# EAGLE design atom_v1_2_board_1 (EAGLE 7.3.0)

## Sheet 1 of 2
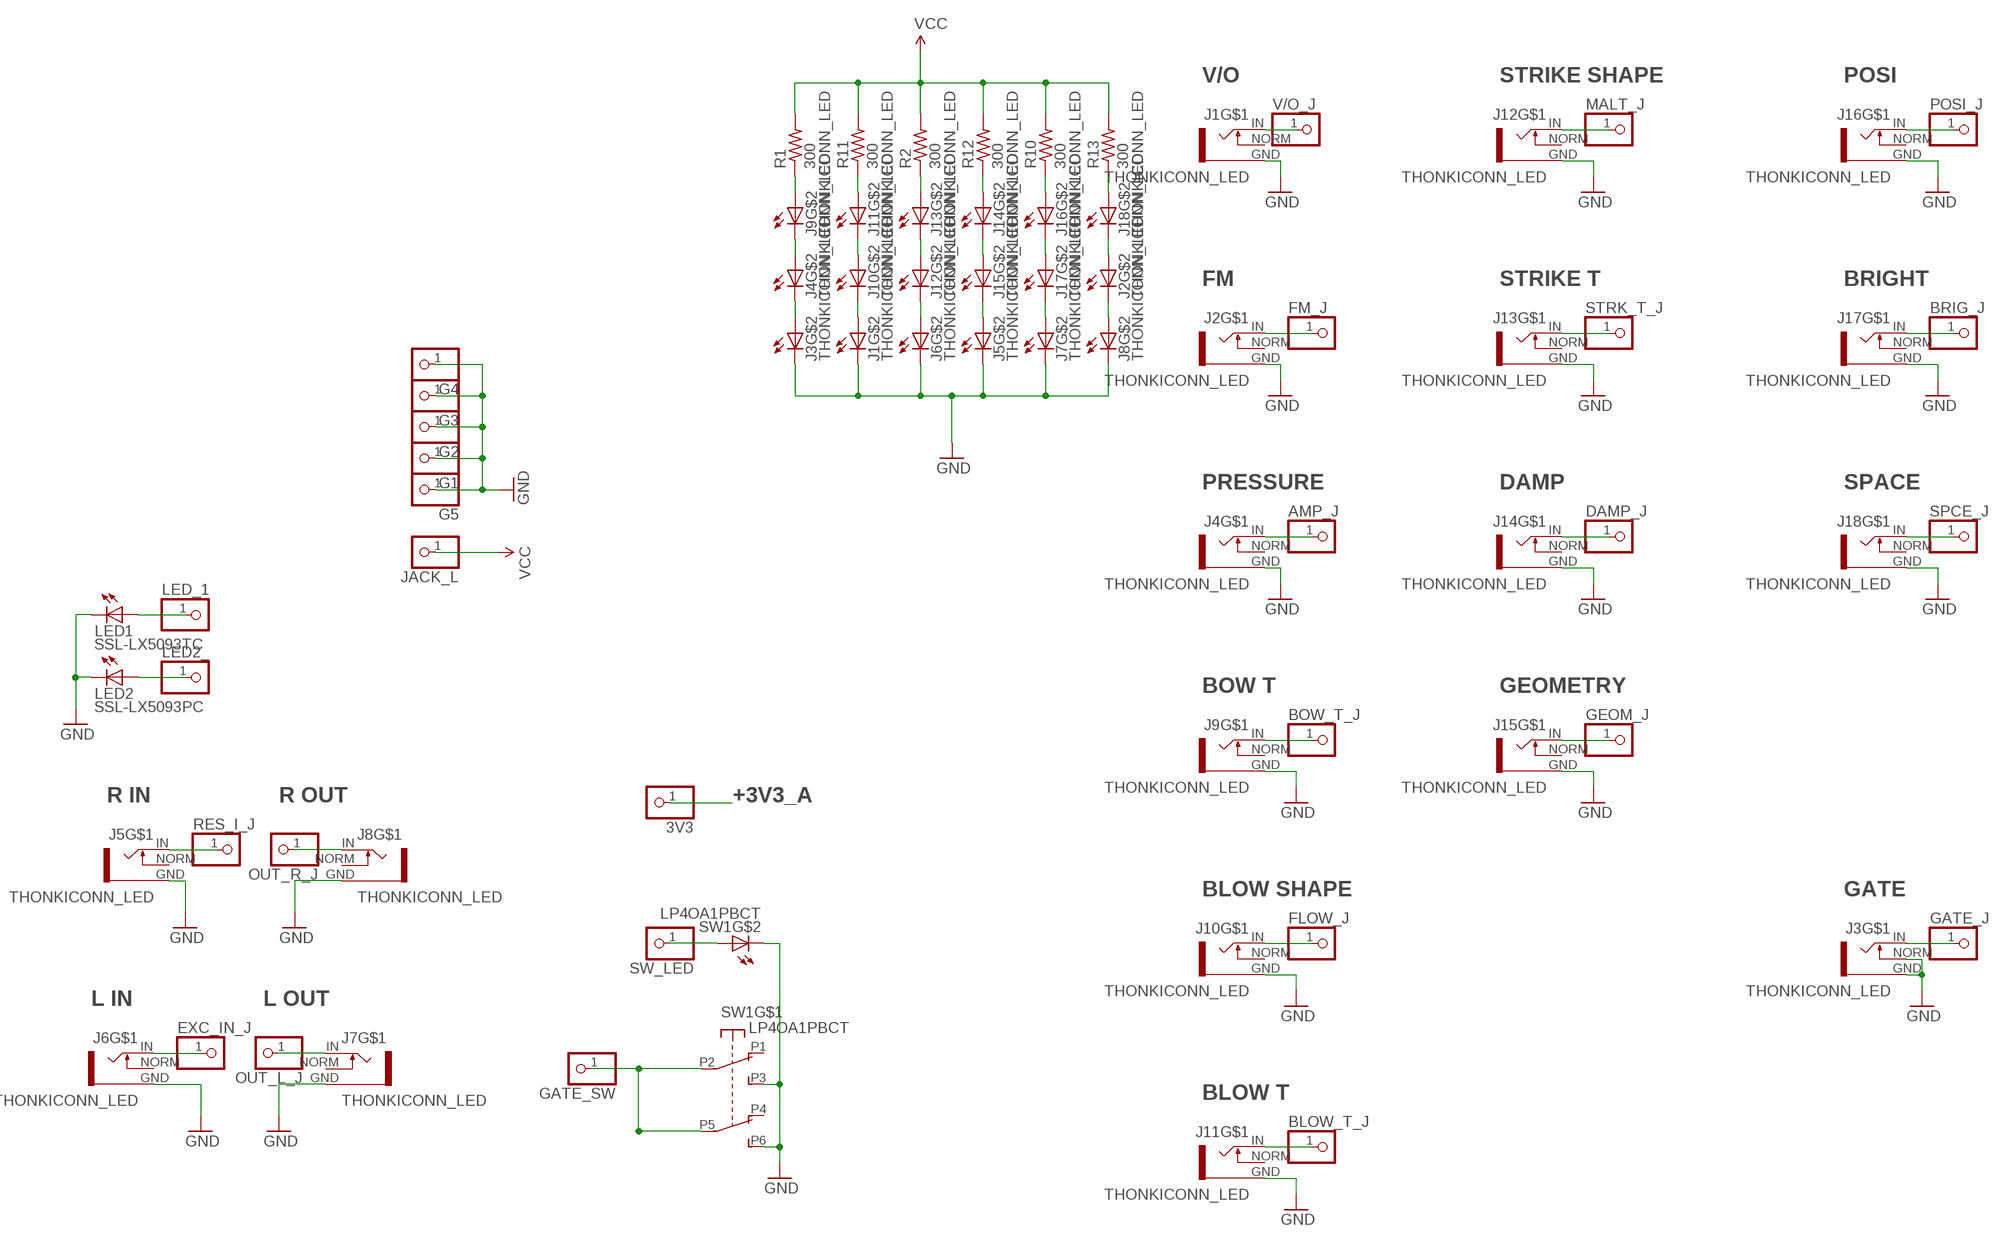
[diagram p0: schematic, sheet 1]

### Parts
3V3  PINHD-1X1  [1X01]
AMP_J  PINHD-1X1  [1X01]
BLOW_T_J  PINHD-1X1  [1X01]
BOW_T_J  PINHD-1X1  [1X01]
BRIG_J  PINHD-1X1  [1X01]
DAMP_J  PINHD-1X1  [1X01]
EXC_IN_J  PINHD-1X1  [1X01]
FLOW_J  PINHD-1X1  [1X01]
FM_J  PINHD-1X1  [1X01]
G1  PINHD-1X1  [1X01]
G2  PINHD-1X1  [1X01]
G3  PINHD-1X1  [1X01]
G4  PINHD-1X1  [1X01]
G5  PINHD-1X1  [1X01]
GATE_J  PINHD-1X1  [1X01]
GATE_SW  PINHD-1X1  [1X01]
GEOM_J  PINHD-1X1  [1X01]
J1  THONKICONN_LED  [LED_JACK]
J2  THONKICONN_LED  [LED_JACK]
J3  THONKICONN_LED  [LED_JACK]
J4  THONKICONN_LED  [LED_JACK]
J5  THONKICONN_LED  [LED_JACK]
J6  THONKICONN_LED  [LED_JACK]
J7  THONKICONN_LED  [LED_JACK]
J8  THONKICONN_LED  [LED_JACK]
J9  THONKICONN_LED  [LED_JACK]
J10  THONKICONN_LED  [LED_JACK]
J11  THONKICONN_LED  [LED_JACK]
J12  THONKICONN_LED  [LED_JACK]
J13  THONKICONN_LED  [LED_JACK]
J14  THONKICONN_LED  [LED_JACK]
J15  THONKICONN_LED  [LED_JACK]
J16  THONKICONN_LED  [LED_JACK]
J17  THONKICONN_LED  [LED_JACK]
J18  THONKICONN_LED  [LED_JACK]
JACK_L  PINHD-1X1  [1X01]
LED1  SSL-LX5093TC  LED5MM  [LED_5MM]
LED2  SSL-LX5093PC  LED5MM  [LED_5MM]
LED2_  PINHD-1X1  [1X01]
LED_1  PINHD-1X1  [1X01]
MALT_J  PINHD-1X1  [1X01]
OUT_L_J  PINHD-1X1  [1X01]
OUT_R_J  PINHD-1X1  [1X01]
POSI_J  PINHD-1X1  [1X01]
R1  300  RESISTOR  [RESISTOR_0603]
R2  300  RESISTOR  [RESISTOR_0603]
R10  300  RESISTOR  [RESISTOR_0603]
R11  300  RESISTOR  [RESISTOR_0603]
R12  300  RESISTOR  [RESISTOR_0603]
R13  300  RESISTOR  [RESISTOR_0603]
RES_I_J  PINHD-1X1  [1X01]
SPCE_J  PINHD-1X1  [1X01]
STRK_T_J  PINHD-1X1  [1X01]
SW1  LP4OA1PBCT  [LP4OA1PBCT]
SW_LED  PINHD-1X1  [1X01]
V/O_J  PINHD-1X1  [1X01]

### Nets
+3V3_A: 3V3.1 ; also sheet 2
GND: G1.1 G2.1 G3.1 G4.1 G5.1 J1.C J1.GND J2.GND J3.C J3.GND J3.NORM J4.GND J5.C J5.GND J6.C J6.GND J7.C J7.GND J8.C J8.GND J9.GND J10.GND J11.GND J12.GND J13.GND J14.GND J15.GND J16.GND J17.GND J18.GND LED1.K(C) LED2.K(C) SW1.L2 SW1.P3(A3) SW1.P6(B3) ; also sheet 2
N$1: J1.IN V/O_J.1
N$2: J11.A R11.1
N$3: J12.IN MALT_J.1
N$4 [wide]: J9.A R1.1
N$5 [wide]: J4.A J9.C
N$6: FM_J.1 J2.IN
N$7 [wide]: J3.A J4.C
N$8: J10.A J11.C
N$9: J1.A J10.C
N$10: J14.A R12.1
N$11: J14.C J15.A
N$12: J13.IN STRK_T_J.1
N$13: J5.A J15.C
N$14: J18.A R13.1
N$15: J2.A J18.C
N$16: DAMP_J.1 J14.IN
N$17 [wide]: J7.A J17.C
N$18 [wide]: J16.C J17.A
N$19 [wide]: J16.A R10.1
N$20: J5.IN RES_I_J.1
N$21: EXC_IN_J.1 J6.IN
N$22 [wide]: J13.A R2.1
N$23 [wide]: J12.A J13.C
N$24 [wide]: J6.A J12.C
N$25: J2.C J8.A
N$26: AMP_J.1 J4.IN
N$29: J16.IN POSI_J.1
N$34: BRIG_J.1 J17.IN
N$36: GEOM_J.1 J15.IN
N$39: J18.IN SPCE_J.1
N$43: GATE_J.1 J3.IN
N$59: LED1.A LED_1.1
N$60: LED2.A LED2_.1
N$83: J8.IN OUT_R_J.1
N$85: J7.IN OUT_L_J.1
N$90: BOW_T_J.1 J9.IN
N$91: FLOW_J.1 J10.IN
N$92: BLOW_T_J.1 J11.IN
N$128: SW1.L1 SW_LED.1
SW_GATE: GATE_SW.1 SW1.P2(A2) SW1.P5(B2)
VCC [wide]: JACK_L.1 R1.2 R2.2 R10.2 R11.2 R12.2 R13.2
Unconnected: J1.NORM J2.NORM J4.NORM J5.NORM J6.NORM J7.NORM J8.NORM J9.NORM J10.NORM J11.NORM J12.NORM J13.NORM J14.NORM J15.NORM J16.NORM J17.NORM J18.NORM SW1.P1(A1) SW1.P4(B1)

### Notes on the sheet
- V/O | STRIKE SHAPE | POSI
- FM | STRIKE T | BRIGHT
- PRESSURE | DAMP | SPACE
- BOW T | GEOMETRY
- R IN | R OUT
- BLOW SHAPE | GATE
- L IN | L OUT
- BLOW T

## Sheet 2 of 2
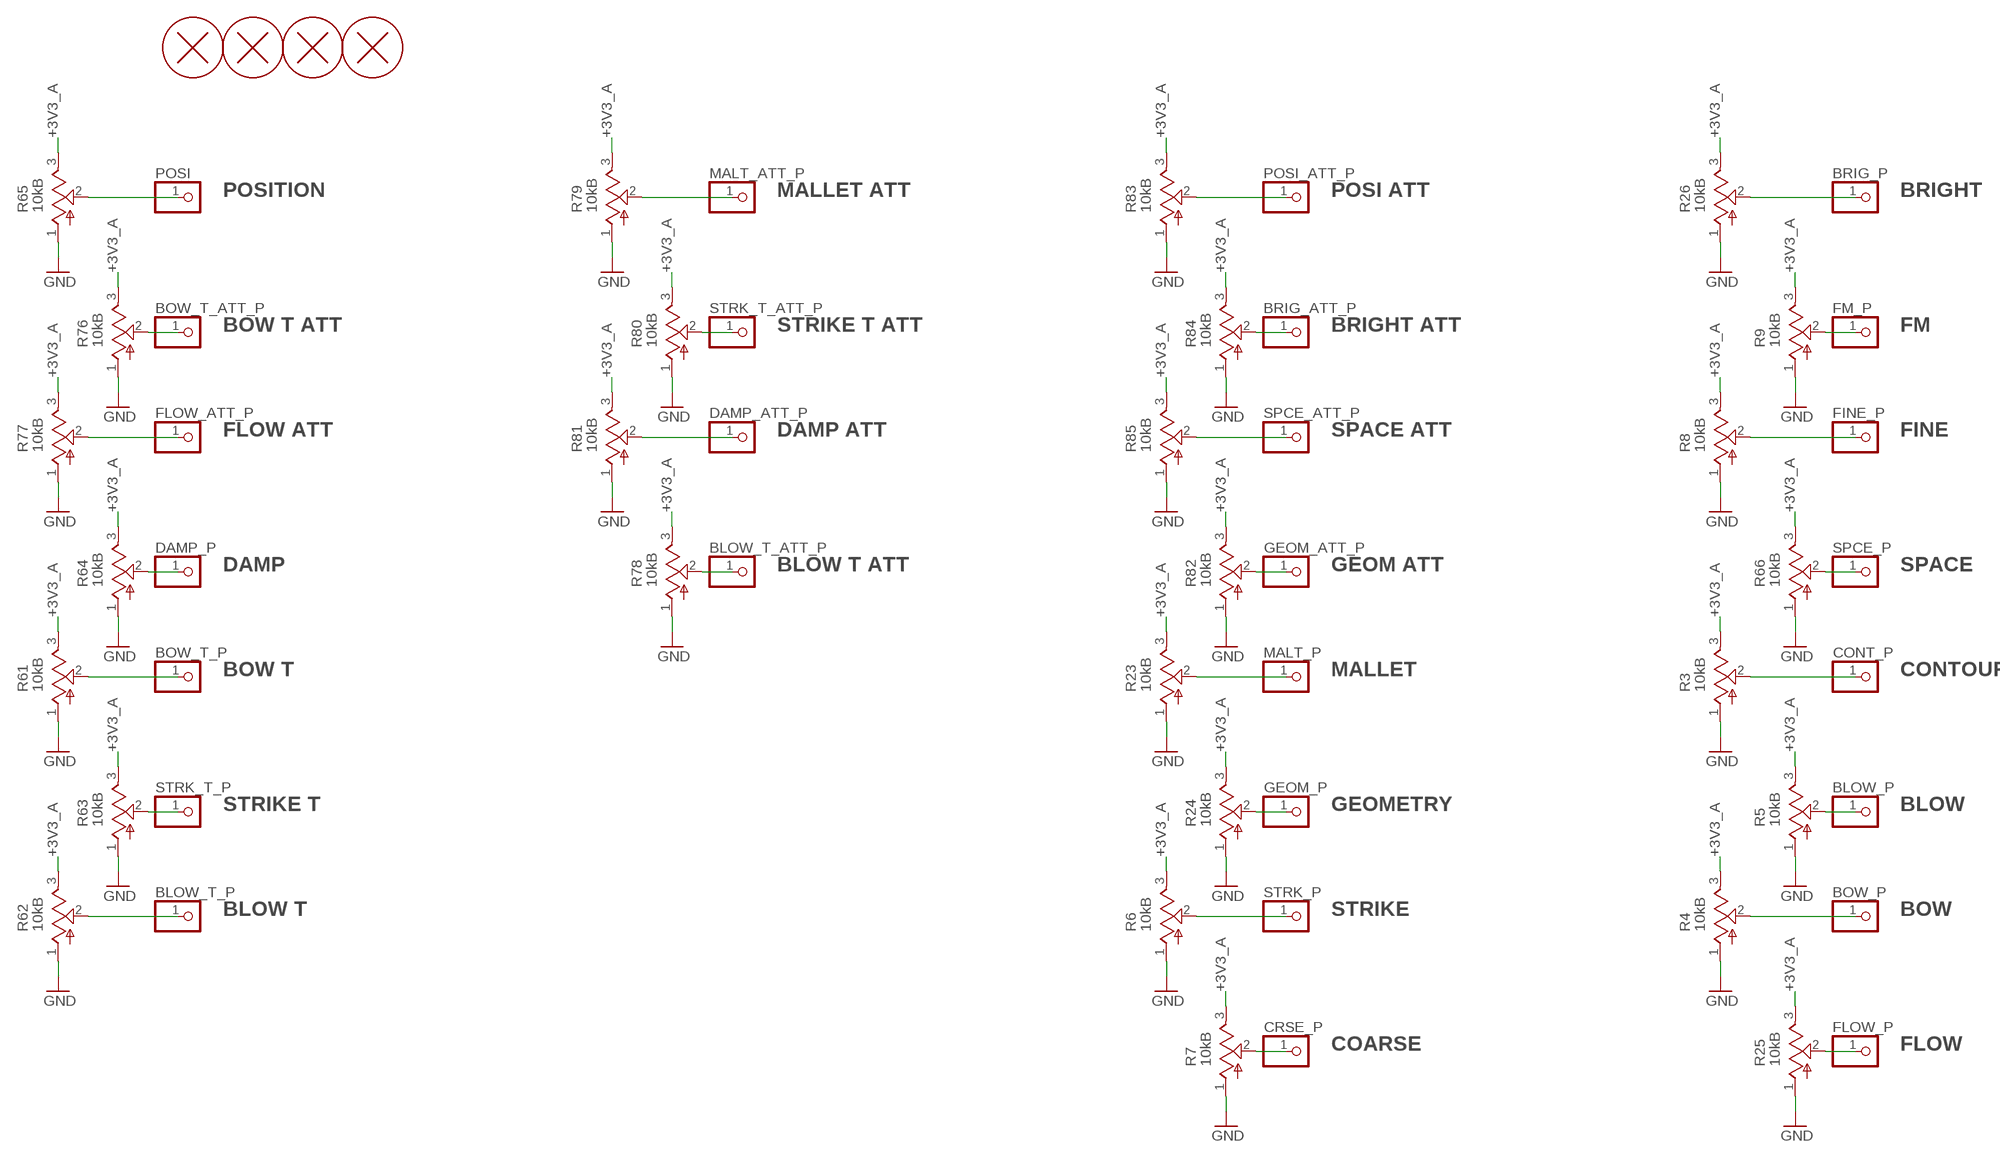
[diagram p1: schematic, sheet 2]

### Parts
BLOW_P  PINHD-1X1  [1X01]
BLOW_T_ATT_P  PINHD-1X1  [1X01]
BLOW_T_P  PINHD-1X1  [1X01]
BOW_P  PINHD-1X1  [1X01]
BOW_T_ATT_P  PINHD-1X1  [1X01]
BOW_T_P  PINHD-1X1  [1X01]
BRIG_ATT_P  PINHD-1X1  [1X01]
BRIG_P  PINHD-1X1  [1X01]
CONT_P  PINHD-1X1  [1X01]
CRSE_P  PINHD-1X1  [1X01]
DAMP_ATT_P  PINHD-1X1  [1X01]
DAMP_P  PINHD-1X1  [1X01]
FINE_P  PINHD-1X1  [1X01]
FLOW_ATT_P  PINHD-1X1  [1X01]
FLOW_P  PINHD-1X1  [1X01]
FM_P  PINHD-1X1  [1X01]
GEOM_ATT_P  PINHD-1X1  [1X01]
GEOM_P  PINHD-1X1  [1X01]
H1  PCB_SCREW  [PCB_SCREW]
H2  PCB_SCREW  [PCB_SCREW]
H3  PCB_SCREW  [PCB_SCREW]
H4  PCB_SCREW  [PCB_SCREW]
MALT_ATT_P  PINHD-1X1  [1X01]
MALT_P  PINHD-1X1  [1X01]
POSI  PINHD-1X1  [1X01]
POSI_ATT_P  PINHD-1X1  [1X01]
R3  10kB  POT_VERTICAL  [ALPS_POT_VERTICAL]
R4  10kB  POT_VERTICAL  [ALPS_POT_VERTICAL]
R5  10kB  POT_VERTICAL  [ALPS_POT_VERTICAL]
R6  10kB  POT_VERTICAL  [ALPS_POT_VERTICAL]
R7  10kB  POT_VERTICAL  [ALPS_POT_VERTICAL]
R8  10kB  POT_VERTICAL  [ALPS_POT_VERTICAL]
R9  10kB  POT_VERTICAL  [ALPS_POT_VERTICAL]
R23  10kB  POT_VERTICAL  [ALPS_POT_VERTICAL]
R24  10kB  POT_VERTICAL  [ALPS_POT_VERTICAL]
R25  10kB  POT_VERTICAL  [ALPS_POT_VERTICAL]
R26  10kB  POT_VERTICAL  [ALPS_POT_VERTICAL]
R61  10kB  POT_VERTICAL  [ALPS_POT_VERTICAL]
R62  10kB  POT_VERTICAL  [ALPS_POT_VERTICAL]
R63  10kB  POT_VERTICAL  [ALPS_POT_VERTICAL]
R64  10kB  POT_VERTICAL  [ALPS_POT_VERTICAL]
R65  10kB  POT_VERTICAL  [ALPS_POT_VERTICAL]
R66  10kB  POT_VERTICAL  [ALPS_POT_VERTICAL]
R76  10kB  POT_VERTICAL  [ALPS_POT_VERTICAL]
R77  10kB  POT_VERTICAL  [ALPS_POT_VERTICAL]
R78  10kB  POT_VERTICAL  [ALPS_POT_VERTICAL]
R79  10kB  POT_VERTICAL  [ALPS_POT_VERTICAL]
R80  10kB  POT_VERTICAL  [ALPS_POT_VERTICAL]
R81  10kB  POT_VERTICAL  [ALPS_POT_VERTICAL]
R82  10kB  POT_VERTICAL  [ALPS_POT_VERTICAL]
R83  10kB  POT_VERTICAL  [ALPS_POT_VERTICAL]
R84  10kB  POT_VERTICAL  [ALPS_POT_VERTICAL]
R85  10kB  POT_VERTICAL  [ALPS_POT_VERTICAL]
SPCE_ATT_P  PINHD-1X1  [1X01]
SPCE_P  PINHD-1X1  [1X01]
STRK_P  PINHD-1X1  [1X01]
STRK_T_ATT_P  PINHD-1X1  [1X01]
STRK_T_P  PINHD-1X1  [1X01]

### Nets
+3V3_A: R3.3(B) R4.3(B) R5.3(B) R6.3(B) R7.3(B) R8.3(B) R9.3(B) R23.3(B) R24.3(B) R25.3(B) R26.3(B) R61.3(B) R62.3(B) R63.3(B) R64.3(B) R65.3(B) R66.3(B) R76.3(B) R77.3(B) R78.3(B) R79.3(B) R80.3(B) R81.3(B) R82.3(B) R83.3(B) R84.3(B) R85.3(B) ; also sheet 1
GND: R3.1(A) R4.1(A) R5.1(A) R6.1(A) R7.1(A) R8.1(A) R9.1(A) R23.1(A) R24.1(A) R25.1(A) R26.1(A) R61.1(A) R62.1(A) R63.1(A) R64.1(A) R65.1(A) R66.1(A) R76.1(A) R77.1(A) R78.1(A) R79.1(A) R80.1(A) R81.1(A) R82.1(A) R83.1(A) R84.1(A) R85.1(A) ; also sheet 1
N$45: BOW_T_ATT_P.1 R76.2(W)
N$46: POSI.1 R65.2(W)
N$47: MALT_ATT_P.1 R79.2(W)
N$48: DAMP_P.1 R64.2(W)
N$49: BOW_T_P.1 R61.2(W)
N$50: R80.2(W) STRK_T_ATT_P.1
N$51: BLOW_T_ATT_P.1 R78.2(W)
N$52: R63.2(W) STRK_T_P.1
N$53: BLOW_T_P.1 R62.2(W)
N$55: FLOW_ATT_P.1 R77.2(W)
N$57: DAMP_ATT_P.1 R81.2(W)
N$58: R85.2(W) SPCE_ATT_P.1
N$62: BRIG_P.1 R26.2(W)
N$63: FINE_P.1 R8.2(W)
N$65: GEOM_ATT_P.1 R82.2(W)
N$67: CRSE_P.1 R7.2(W)
N$68: FM_P.1 R9.2(W)
N$69: R6.2(W) STRK_P.1
N$70: GEOM_P.1 R24.2(W)
N$71: MALT_P.1 R23.2(W)
N$72: FLOW_P.1 R25.2(W)
N$73: BOW_P.1 R4.2(W)
N$74: CONT_P.1 R3.2(W)
N$75: BLOW_P.1 R5.2(W)
N$76: POSI_ATT_P.1 R83.2(W)
N$77: BRIG_ATT_P.1 R84.2(W)
N$78: R66.2(W) SPCE_P.1

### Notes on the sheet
- POSITION | MALLET ATT | POSI ATT | BRIGHT
- BOW T ATT | STRIKE T ATT | BRIGHT ATT | FM
- FLOW ATT | DAMP ATT | SPACE ATT | FINE
- DAMP | BLOW T ATT | GEOM ATT | SPACE
- BOW T | MALLET | CONTOUR
- STRIKE T | GEOMETRY | BLOW
- BLOW T | STRIKE | BOW
- COARSE | FLOW

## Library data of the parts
3V3 AMP_J BLOW_P BLOW_T_ATT_P BLOW_T_J BLOW_T_P BOW_P BOW_T_ATT_P BOW_T_J BOW_T_P BRIG_ATT_P BRIG_J BRIG_P CONT_P CRSE_P DAMP_ATT_P DAMP_J DAMP_P EXC_IN_J FINE_P FLOW_ATT_P FLOW_J FLOW_P FM_J FM_P G1-G5 GATE_J GATE_SW GEOM_ATT_P GEOM_J GEOM_P JACK_L LED2_ LED_1 MALT_ATT_P MALT_J MALT_P OUT_L_J OUT_R_J POSI POSI_ATT_P POSI_J RES_I_J SPCE_ATT_P SPCE_J SPCE_P STRK_P STRK_T_ATT_P STRK_T_J STRK_T_P SW_LED V/O_J = parts_aman:PINHD-1X1: PIN HEADER
H1-H4 = parts_aman:PCB_SCREW
J1-J18 = parts_aman:THONKICONN_LED
LED1 LED2 = parts_aman:LED
R1 R2 R10-R13 = parts_aman:RESISTOR
R3-R9 R23-R26 R61-R66 R76-R85 = parts_aman:POT_VERTICAL
SW1 = og-switch:LP4OA1PBCT

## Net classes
0 default: width 0.152 mm, drill 0.305 mm, clearance 0.152 mm
1 wide: width 0.305 mm, drill 0.305 mm, clearance 0.305 mm

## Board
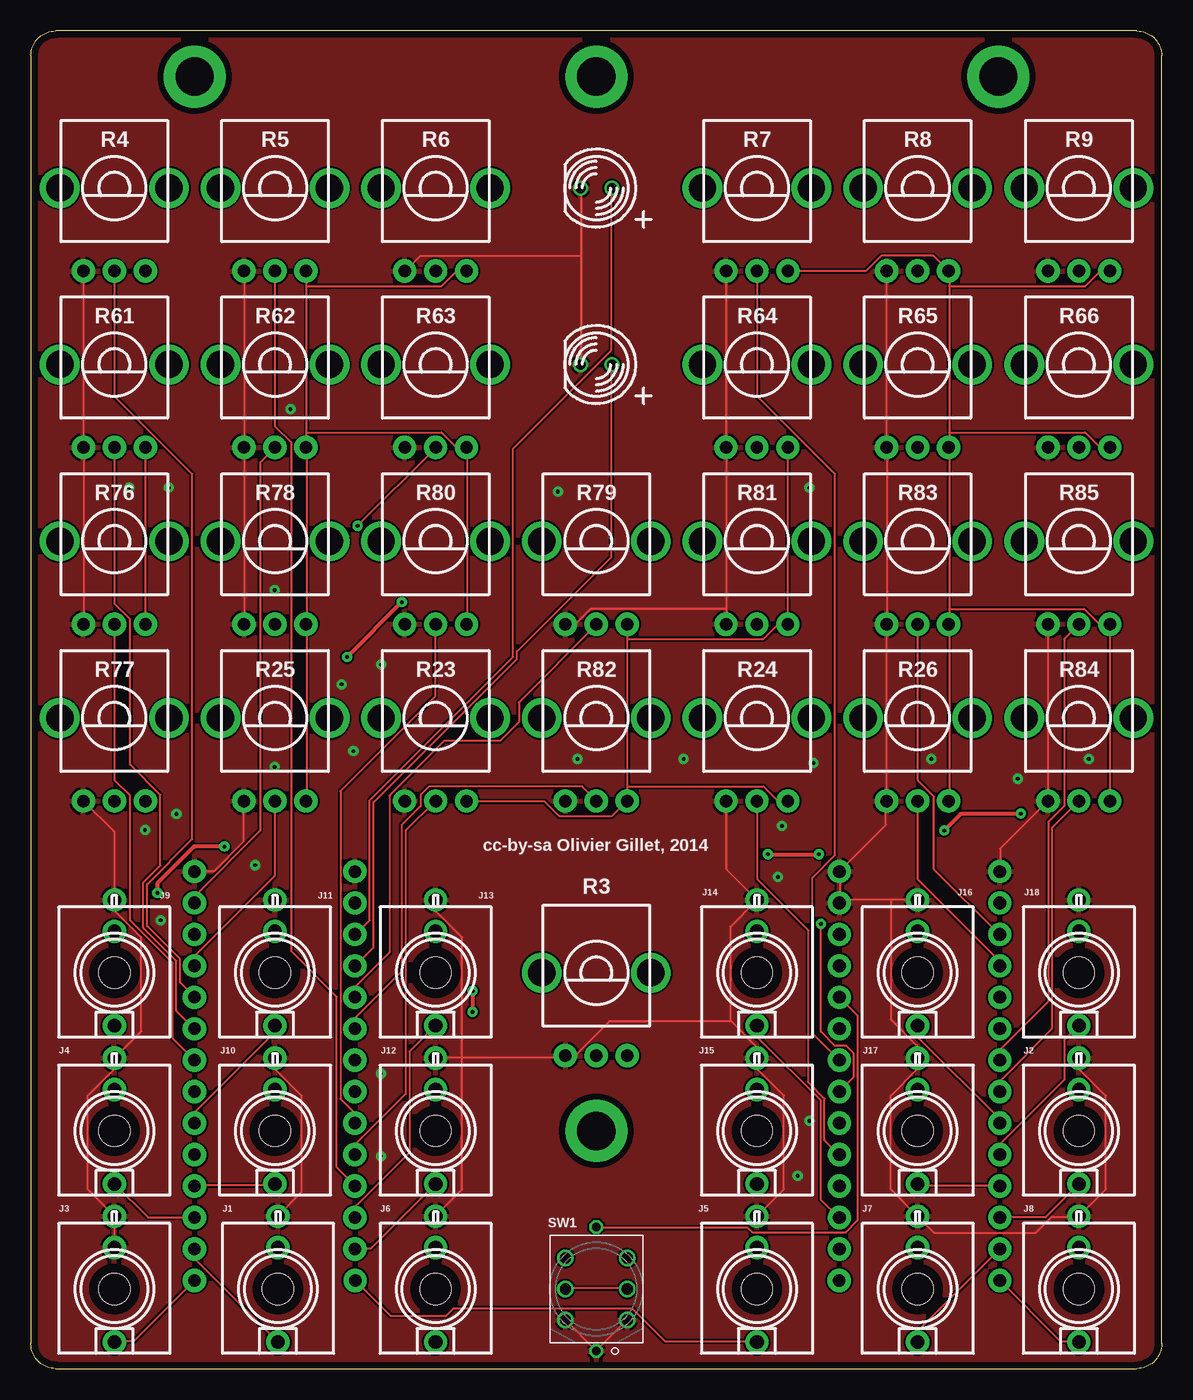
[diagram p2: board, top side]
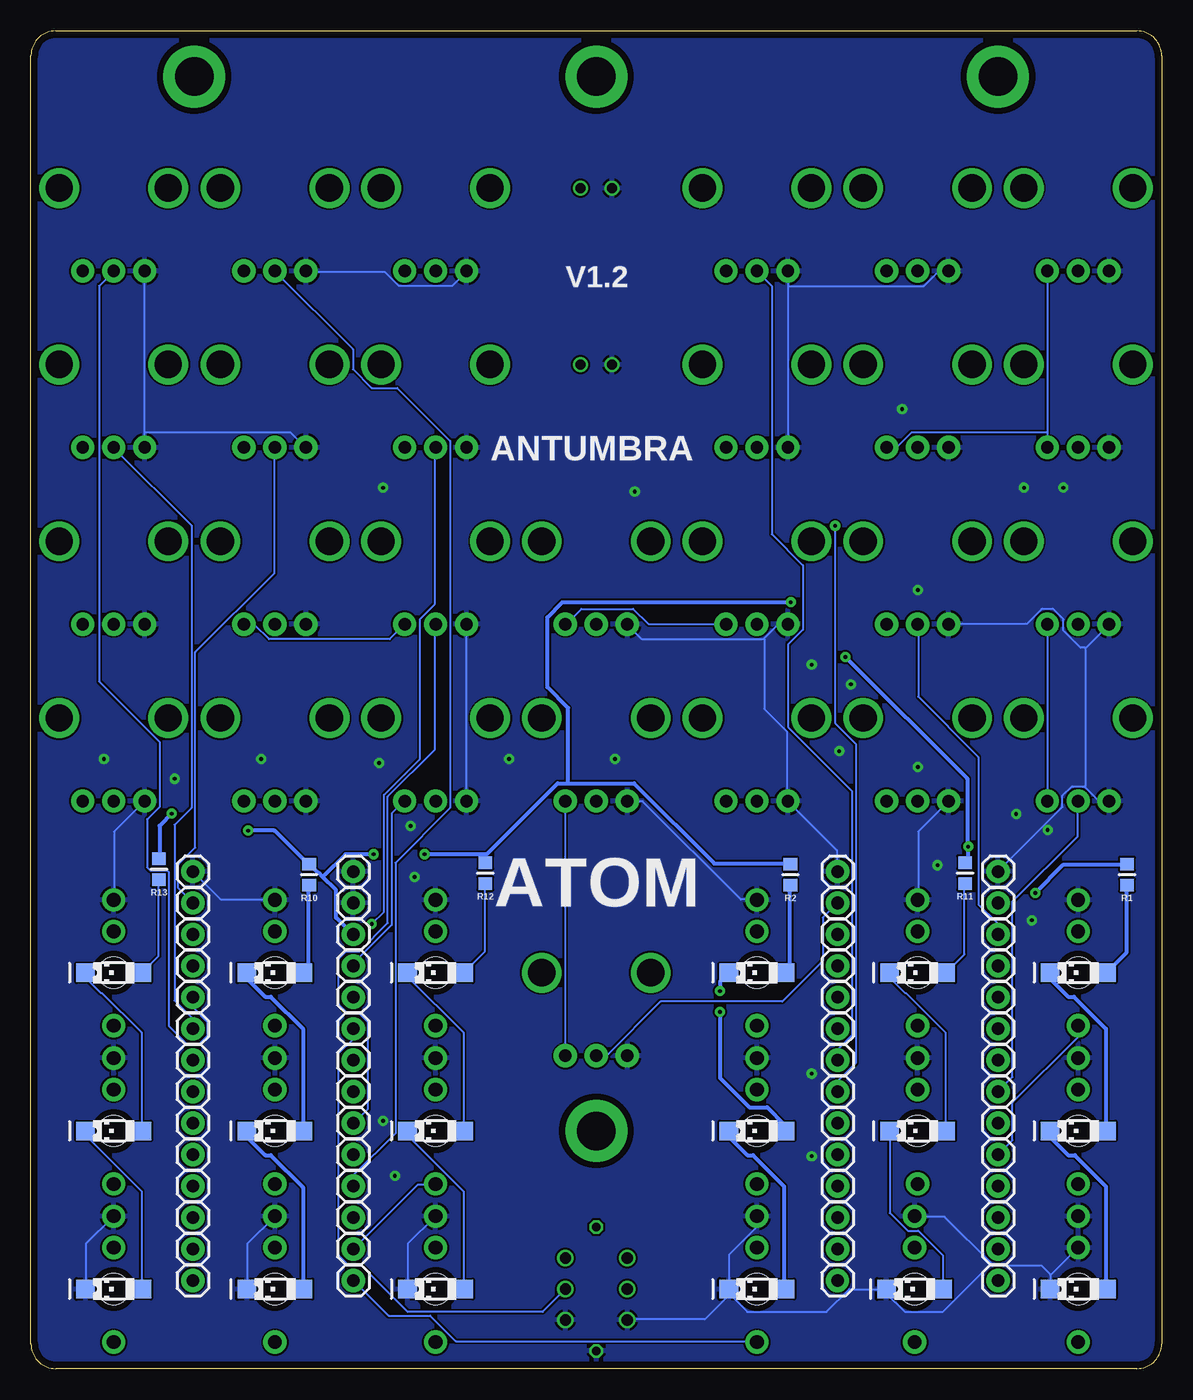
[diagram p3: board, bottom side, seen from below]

Size 91.3 x 108 mm. Coordinates in mm from the lower left corner, seen from the top.
Outline: 2,0 89.3,0 arc90 91.3,2 91.3,106 arc90 89.3,108 2,108 arc90 0,106 0,2 arc90 2,0
Copper layers (1*16): Top 0.035mm / dielectric 1.5mm / Bottom 0.035mm
Design rules "PCBCart-Standard": minimum track width 6mil, minimum drill 12mil, track to track 6mil, track to pad 6mil, pad to pad 6mil, via to via 6mil, smd to smd 6mil, copper to edge 20mil, drill to drill 8mil, minimum pad ring 8mil, minimum via ring 10mil, stop-mask expansion 3mil, vias tented up to drill 25mil, thermal gap 8mil

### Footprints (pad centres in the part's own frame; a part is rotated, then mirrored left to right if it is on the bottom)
1X01 = drill 1.016 pad 1.88: 1 0,0
PCB_SCREW = drill 3.1 pad 5: P$1 0,0
LED_JACK = smd 1.5 x 1.5 bottom: A 2.266,0; C -2.266,0 | drill 1.1 pad 1.88: GND 0,-5.88; IN 0,4.28; NORM 0,-3.34 | hole 2.5: 0,0
LED_5MM = drill 0.813: A -1.27,0; K 1.27,0
RESISTOR_0603 = smd 1 x 1.1: 1 -0.85,0; 2 0.85,0
ALPS_POT_VERTICAL = drill 1 pad 1.88: 1 -2.5,-6.7; 2 0,-6.7; 3 2.5,-6.7 | drill 2.2 pad 3.175: P$4 4.4,0; P$5 -4.4,0
LP4OA1PBCT = drill 0.7 octagon: L1 5,0; L2 -5,0 | drill 0.9: P1 2.5,2.5; P2 0,2.5; P3 -2.5,2.5; P4 2.5,-2.5; P5 0,-2.5; P6 -2.5,-2.5

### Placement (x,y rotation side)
3V3  65.28,32.51 0 bottom
AMP_J  13.21,12.19 0 bottom
BLOW_P  26.16,14.73 0 bottom
BLOW_T_ATT_P  13.21,35.05 0 bottom
BLOW_T_J  13.21,19.81 0 bottom
BLOW_T_P  13.21,37.59 0 bottom
BOW_P  13.21,29.97 0 bottom
BOW_T_ATT_P  13.21,24.89 0 bottom
BOW_T_J  13.21,17.27 0 bottom
BOW_T_P  13.21,27.43 0 bottom
BRIG_ATT_P  78.23,22.35 0 bottom
BRIG_J  78.23,14.73 0 bottom
BRIG_P  78.23,32.51 0 bottom
CONT_P  26.16,37.59 0 bottom
CRSE_P  65.28,24.89 0 bottom
DAMP_ATT_P  65.28,19.81 0 bottom
DAMP_J  65.28,12.19 0 bottom
DAMP_P  65.28,22.35 0 bottom
EXC_IN_J  65.26,7.11 0 bottom
FINE_P  65.28,14.73 0 bottom
FLOW_ATT_P  13.21,22.35 0 bottom
FLOW_J  13.21,14.73 0 bottom
FLOW_P  13.21,32.51 0 bottom
FM_J  78.23,12.19 0 bottom
FM_P  78.23,29.97 0 bottom
G1  13.21,40.13 0 bottom
G2  26.16,40.13 0 bottom
G3  65.28,40.13 0 bottom
G4  78.23,40.13 0 bottom
G5  65.28,37.59 0 bottom
GATE_J  13.21,7.11 0 bottom
GATE_SW  65.28,27.43 0 bottom
GEOM_ATT_P  26.16,27.43 0 bottom
GEOM_J  65.28,9.65 0 bottom
GEOM_P  65.28,17.27 0 bottom
H1  13.22,104.31 0 top
H2  78.12,104.31 0 top
H3  45.65,104.31 0 top
H4  45.65,19.19 0 top
J1  19.94,6.42 180 top
J2  84.62,19.19 180 top
J3  6.74,6.42 180 top
J4  6.74,19.19 180 top
J5  58.62,6.42 180 top
J6  32.68,6.42 180 top
J7  71.6,6.42 180 top
J8  84.62,6.42 180 top
J9  6.74,31.96 180 top
J10  19.7,19.19 180 top
J11  19.7,31.96 180 top
J12  32.68,19.19 180 top
J13  32.68,31.96 180 top
J14  58.62,31.96 180 top
J15  58.62,19.19 180 top
J16  71.6,31.96 180 top
J17  71.6,19.19 180 top
J18  84.62,31.96 180 top
JACK_L  65.28,35.05 0 bottom
LED1  45.65,95.32 180 top
LED2  45.65,81.07 180 top
LED2_  26.16,32.51 0 bottom
LED_1  26.16,35.05 0 bottom
MALT_ATT_P  26.16,29.97 0 bottom
MALT_J  26.16,9.65 0 bottom
MALT_P  26.16,17.27 0 bottom
OUT_L_J  78.23,9.65 0 bottom
OUT_R_J  78.23,7.11 0 bottom
POSI  78.23,37.59 0 bottom
POSI_ATT_P  78.23,35.05 0 bottom
POSI_J  78.23,19.81 0 bottom
R1  2.79,39.88 90 bottom
R2  29.97,39.88 90 bottom
R3  45.65,31.96 0 top
R4  6.74,95.32 0 top
R5  19.7,95.32 0 top
R6  32.68,95.32 0 top
R7  58.62,95.32 0 top
R8  71.6,95.32 0 top
R9  84.62,95.32 0 top
R10  68.83,39.88 90 bottom
R11  15.88,40.01 90 bottom
R12  54.61,40.01 90 bottom
R13  80.96,40.32 90 bottom
R23  32.68,52.52 0 top
R24  58.62,52.52 0 top
R25  19.7,52.52 0 top
R26  71.6,52.52 0 top
R61  6.74,81.07 0 top
R62  19.7,81.07 0 top
R63  32.68,81.07 0 top
R64  58.62,81.07 0 top
R65  71.6,81.07 0 top
R66  84.62,81.07 0 top
R76  6.74,66.8 0 top
R77  6.74,52.52 0 top
R78  19.7,66.8 0 top
R79  45.65,66.8 0 top
R80  32.68,66.8 0 top
R81  58.62,66.8 0 top
R82  45.65,52.52 0 top
R83  71.6,66.8 0 top
R84  84.62,52.52 0 top
R85  84.62,66.8 0 top
RES_I_J  26.18,7.11 0 bottom
SPCE_ATT_P  78.23,24.89 0 bottom
SPCE_J  78.23,17.27 0 bottom
SPCE_P  78.23,27.43 0 bottom
STRK_P  26.16,24.89 0 bottom
STRK_T_ATT_P  26.16,19.81 0 bottom
STRK_T_J  26.16,12.19 0 bottom
STRK_T_P  26.16,22.35 0 bottom
SW1  45.65,6.42 90 top
SW_LED  65.28,29.97 0 bottom
V/O_J  13.21,9.65 0 bottom

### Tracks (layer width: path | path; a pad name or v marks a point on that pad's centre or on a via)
+3V3_A
  Top 0.152: R84.3 87.1,45.87 87.1,60.05 R85.3 87.02,60.05 86.33,60.05 85.04,61.34 74.14,61.34 | R26.3 74.14,45.87 74.14,60.05 R83.3 74.14,60.12 74.14,61.34 | 74.14,87.4 74.14,88.54 R8.3 74.07,88.62 72.85,89.84 68.66,89.84 67.44,88.62 61.19,88.62 R7.3 | 74.14,87.4 74.14,75.59 | 74.14,75.59 74.14,74.37 R65.3 74.14,74.3 74.14,61.34 | 74.14,75.59 85.11,75.59 86.33,74.37 87.1,74.37 R66.3 | 74.14,87.4 85.11,87.4 86.26,88.54 87.1,88.54 R9.3 | R25.3 22.25,45.87 22.25,60.05 R78.3 22.25,60.12 22.25,74.3 R62.3 22.25,74.37 22.25,75.59 | R80.3 35.2,60.12 35.2,74.3 R63.3 35.13,74.37 34.37,74.37 33.15,75.59 22.25,75.59 | 22.25,75.59 22.25,87.4 | 22.25,87.4 22.25,88.54 R5.3 | 22.25,87.4 33.15,87.4 34.29,88.54 35.13,88.54 R6.3 | R76.3 9.22,60.12 9.22,74.3 R61.3 | R23.3 35.2,45.8 41.45,45.8 42.67,44.58 46.86,44.58 48.08,45.8 R82.3 48.16,45.87 48.16,47.02 | 48.16,47.02 48.16,58.9 | 48.16,58.9 48.16,60.05 R79.3 | 48.16,47.02 59.13,47.02 60.27,45.87 61.11,45.87 R24.3 | 48.16,58.9 59.13,58.9 60.27,60.05 61.11,60.05 R81.3 61.11,60.12 61.11,74.3 R64.3
  Bottom 0.152: R77.3 9.22,45.87 9.22,60.05 R76.3 | 9.22,75.59 9.22,88.54 R4.3 | 9.22,75.59 9.22,74.37 R61.3 | 9.22,75.59 20.19,75.59 21.41,74.37 22.17,74.37 R62.3 | R3.3 48.16,25.3 48.16,45.8 R82.3 | 3V3.1 65.23,32.54 65.23,32.77 62.18,35.81 62.18,44.81 61.19,45.8 R24.3 | R80.3 35.2,60.12 41.45,60.12 42.67,61.34 46.86,61.34 48.08,60.12 R79.3 | R83.3 74.07,60.05 73.23,60.05 72.08,58.9 62.33,58.9 61.19,60.05 R81.3
GND  (via drill 0.3)
  Top 0.152: R8.1 69.11,88.54 69.11,74.45 R65.1 69.11,74.3 69.11,60.12 R83.1 69.11,60.05 69.11,45.87 R26.1 69.04,45.8 69.04,43.89 G3.1 65.3,40.08 65.3,37.87 | J2.GND 84.66,24.99 84.66,24.16 86.79,22.02 86.79,14.48 84.66,12.34 J8.GND 84.58,12.27 82.45,12.27 81.15,10.97 72.92,10.97 71.63,12.27 J7.GND 71.55,12.34 69.42,14.48 69.42,22.02 71.55,24.16 71.55,24.99 J17.GND 71.55,25.07 71.55,26.06 69.42,28.19 69.42,37.87 | 65.3,37.87 65.3,37.64 G5.1 65.3,37.87 | 65.3,37.87 69.42,37.87 | 69.42,37.87 71.55,37.87 J16.GND | G4.1 78.26,40.16 78.26,41.99 82.07,45.8 R84.1 82.14,45.87 82.14,60.05 R85.1 | R78.1 17.22,60.12 17.22,74.3 R62.1 17.22,74.45 17.22,88.54 R5.1 | 44.42,89.84 44.42,95.25 LED1.K | 44.42,89.84 44.42,81.08 LED2.K | 44.42,89.84 31.47,89.84 30.25,88.62 R6.1 | R77.1 4.27,45.8 6.71,43.36 6.71,37.87 J9.GND 6.78,37.8 6.78,36.96 8.91,34.82 8.91,27.2 6.78,25.07 J4.GND 6.71,24.99 6.71,24.16 4.57,22.02 4.57,14.48 6.71,12.34 J3.GND 6.78,12.27 6.78,9.83 J3.NORM | G1.1 13.26,40.16 14.78,40.16 17.14,42.52 17.14,45.8 R25.1 | R76.1 4.27,60.12 4.27,74.3 R61.1 4.27,74.37 4.27,88.54 R4.1 | 34.82,25.07 42.98,25.07 43.13,25.22 R3.1 43.2,25.3 43.97,25.3 46.71,28.04 56.46,28.04 56.5,28.08 | 34.82,25.07 J12.GND | 34.82,25.07 34.82,34.82 32.69,36.96 32.69,37.8 J13.GND | J10.GND 19.74,24.99 19.74,24.16 21.87,22.02 21.87,14.25 19.96,12.34 J1.GND | 45.64,1.45 43.2,3.89 SW1.P3 | 45.64,1.45 48.08,3.89 SW1.P6 | 45.64,1.45 SW1.L2 | 34.82,25.07 34.82,14.48 32.69,12.34 J6.GND | J5.GND 58.67,12.34 60.81,14.48 60.81,22.02 58.67,24.16 58.67,24.99 J15.GND 58.6,25.07 58.6,25.98 56.5,28.08
  Top 0.152: R24.1 56.16,45.8 56.16,40.31 58.6,37.87 J14.GND 58.6,37.8 56.46,35.66 56.46,28.12 56.5,28.08 | 56.16,61.34 56.16,74.3 R64.1 56.16,74.37 56.16,88.54 R7.1 | 56.16,61.34 56.16,60.12 R81.1 | 56.16,61.34 45.19,61.34 43.97,60.12 43.2,60.12 R79.1
  Bottom 0.152: 82.14,75.59 82.14,88.54 R9.1 | 82.14,75.59 82.14,74.37 R66.1 | 82.14,75.59 70.33,75.59 69.11,74.37 R65.1 | J8.C 86.87,6.48 86.87,10.06 84.66,12.27 J8.GND | J7.C 73.84,6.48 73.84,10.06 71.63,12.27 J7.GND | J18.GND 84.58,37.87 84.58,43.36 82.14,45.8 R84.1 | G4.1 75.97,37.87 71.63,37.87 J16.GND | 30.18,87.4 30.18,88.54 R6.1 | 30.18,87.4 R63.1 | 30.18,87.4 19.2,87.4 18.06,88.54 17.22,88.54 R5.1 | J11.GND 19.66,37.87 19.66,43.36 17.22,45.8 R25.1 | 6.21,46.98 6.25,47.02 7.24,47.02 8,46.25 8,45.34 G1.1 | 6.21,46.98 5.11,45.87 4.27,45.87 R77.1 | 6.13,58.18 4.27,60.05 R76.1 | 6.13,58.18 6.17,58.14 6.17,47.02 6.21,46.98 | R78.1 17.14,60.12 10.9,60.12 9.68,61.34 8.76,61.34 7.92,60.5 7.92,59.59 6.55,58.22 6.17,58.22 6.13,58.18 | R82.1 43.13,45.8 41.91,45.8 33.98,37.87 32.69,37.87 J13.GND | 8.95,7.58 6.78,9.75 J3.NORM | 8.95,7.58 8.99,7.54 8.99,6.48 J3.C | 13.75,8.5 13.56,8.31 9.68,8.31 8.95,7.58 | 13.75,8.5 17.53,12.27 19.89,12.27 J1.GND | J6.C 34.9,6.4 34.9,6.02 33.45,4.57 27.05,4.57 25.22,6.4 22.25,6.4 J1.C 22.25,6.33 22.25,6.1 20.73,4.57 17.68,4.57 13.75,8.5 | J6.GND 32.69,12.27 32.69,11.43 34.9,9.22 34.9,6.48 J6.C | SW1.P3 43.13,3.96 36.88,3.96 34.9,5.94 J6.C | G2.1 26.21,40.16 26.21,41.83 30.18,45.8 R23.1 30.25,45.87 30.25,51.44 32.08,53.26 32.08,58.9 32.12,58.94 | 32.12,58.94 32.16,58.9 41.99,58.9 43.13,60.05 R79.1 | 32.12,58.94 31.01,60.05 30.25,60.05 R80.1 | J5.C 60.88,6.48 60.88,10.06 58.67,12.27 J5.GND | R24.1 56.16,45.87 56.16,60.05 R81.1 | R8.1 69.04,88.54 62.71,88.54 61.57,87.4 57.3,87.4 56.16,88.54 R7.1
  other vias: 11.75,44.77 9.21,43.5 18.1,40.64 26.04,49.85 28.26,56.83 42.55,70.8 20.95,77.47 85.41,49.21 72.71,49.21 79.69,47.62 63.18,48.9 52.7,49.21 44.13,49.21 60.64,43.81 60.33,39.69 61.91,15.56 28.26,17.14 28.26,23.81 10.48,36.2 19.68,48.58 19.68,62.87 25.08,55.24 11.11,71.12 7.94,71.12 62.87,71.12 62.87,20
  pour Bottom: 0,0 91.3,0 91.3,108 0,108
  pour Top: 0,0 91.3,0 91.3,108 0,108
N$1
  Top 0.152: V/O_J.1 13.26,9.6 13.26,8.84 19.89,2.21 J1.IN
N$2
  Bottom 0.152: R11.1 15.93,39.09 15.93,33.45 17.37,32 J11.A
N$3
  Top 0.152: MALT_J.1 26.21,9.68 27.43,9.68 32.61,14.86 J12.IN
N$4
  Bottom 0.305: R1.1 2.82,39.01 2.82,33.6 4.42,32 J9.A
N$5
  Bottom 0.305: J4.A 4.5,19.2 4.5,27.43 7.09,30.02 7.54,30.02 8.99,31.47 8.99,31.93 J9.C
N$6
  Top 0.152: FM_J.1 81.92,12.19 84.58,14.86 J2.IN
N$7
  Bottom 0.305: J3.A 4.5,6.48 4.5,14.71 7.01,17.22 7.54,17.22 8.99,18.67 8.99,19.13 J4.C
N$8
  Bottom 0.152: J10.A 17.45,19.2 17.45,27.13 20.65,30.33 20.73,30.33 21.95,31.55 21.95,31.93 J11.C
N$9
  Bottom 0.152: J1.A 17.68,6.48 17.68,9.14 19.66,11.12 20.5,11.12 21.95,12.57 21.95,19.13 J10.C
N$10
  Bottom 0.152: R12.1 54.63,39.09 54.63,33.68 56.31,32 J14.A
N$11
  Bottom 0.152: J15.A 56.39,19.2 56.39,27.13 60.88,31.62 60.88,31.93 J14.C
N$12
  Top 0.152: STRK_T_J.1 26.21,12.19 26.21,13.11 30.56,17.45 30.56,25.6 32.61,27.66 J13.IN
N$13
  Bottom 0.152: J5.A 56.39,6.48 56.39,14.33 60.88,18.82 60.88,19.13 J15.C
N$14
  Bottom 0.152: R13.1 81,39.47 81,33.3 82.3,32 J18.A
N$15
  Bottom 0.152: J2.A 82.37,19.2 82.37,27.13 85.57,30.33 85.65,30.33 86.87,31.55 86.87,31.93 J18.C
N$16
  Top 0.152: J14.IN 58.67,27.66 58.67,26.75 63.78,21.64 63.78,13.64 65.23,12.19 DAMP_J.1
N$17
  Bottom 0.305: J7.A 69.34,6.48 69.34,14.63 71.93,17.22 72.39,17.22 73.84,18.67 73.84,19.13 J17.C
N$18
  Bottom 0.305: J17.A 69.34,19.2 69.34,27.43 71.93,30.02 72.39,30.02 73.84,31.47 73.84,31.93 J16.C
N$19
  Bottom 0.305: R10.1 68.89,39.01 68.89,32.38 69.27,32 J16.A
N$20
  Top 0.152: J5.IN 58.6,2.21 51.21,2.21 48.54,4.88 34.14,4.88 33.53,4.27 29.03,4.27 26.21,7.09 RES_I_J.1
N$21
  Bottom 0.152: J6.IN 32.69,2.21 57,2.21 59.05,4.27 62.41,4.27 65.23,7.09 EXC_IN_J.1
N$22
  Bottom 0.305: R2.1 30.02,39.01 30.02,32.38 30.4,32 J13.A
N$23  (via drill 0.3)
  Top 0.305: v35.66,30.48 v35.66,28.8
  Bottom 0.305: v35.66,28.8 35.66,23.47 33.3,21.11 31.85,21.11 30.48,19.74 30.48,19.2 J12.A | v35.66,30.48 35.66,31.24 34.98,31.93 J13.C
N$24
  Bottom 0.305: J6.A 30.48,6.48 30.48,14.71 32.99,17.22 33.45,17.22 34.9,18.67 34.9,19.13 J12.C
N$25
  Bottom 0.152: J8.A 82.37,6.48 82.37,14.33 86.87,18.82 86.87,19.13 J2.C
N$26
  Top 0.152: AMP_J.1 9.45,12.19 6.78,14.86 J4.IN
N$29
  Top 0.152: J16.IN 71.63,27.66 71.63,26.75 78.18,20.19 78.18,19.81 POSI_J.1
N$34
  Top 0.152: BRIG_J.1 78.18,14.78 71.7,14.78 71.63,14.86 J17.IN
N$36
  Bottom 0.152: J15.IN 58.67,14.86 60.05,14.86 65.23,9.68 GEOM_J.1
N$39
  Top 0.152: SPCE_J.1 78.26,17.3 78.26,18.14 83.44,23.32 83.44,26.52 84.58,27.66 J18.IN
N$43
  Top 0.152: GATE_J.1 8.31,2.21 6.78,2.21 J3.IN
N$45
  Top 0.152: BOW_T_ATT_P.1 11.43,26.67 11.43,32.77 8,36.2 8,46.25 6.78,47.47 6.78,60.05 R76.2
N$46
  Bottom 0.152: R65.2 71.63,74.3 71.63,64.24 78.03,57.84 78.03,42.06 79.4,40.69 79.4,38.79 78.26,37.64 POSI.1
N$47
  Top 0.152: MALT_ATT_P.1 26.21,30.02 26.21,30.86 28.96,33.6 28.96,46.25 33.38,50.67 37.87,50.67 39.4,52.2 39.4,53.8 45.64,60.05 R79.2
N$48  (via drill 0.3)
  Top 0.152: v63.78,35.89 63.78,27.2 64.92,26.06 65.84,26.06 66.45,25.45 66.45,23.55 65.3,22.4 DAMP_P.1
  Bottom 0.152: v63.78,35.89 62.79,36.88 62.79,46.33 59.89,49.23 59.89,60.5 58.67,61.72 58.67,74.3 R64.2
N$49
  Top 0.152: R61.2 6.78,74.3 6.78,61.72 8,60.5 8,48.77 10.44,46.33 10.44,40.62 9.07,39.24 9.07,35.59 11.73,32.92 11.73,28.88 13.18,27.43 BOW_T_P.1
N$50
  Top 0.152: STRK_T_ATT_P.1 26.14,19.81 26.14,20.65 24.99,21.79 24.99,46.63 32.61,54.25 32.61,60.05 R80.2
N$51
  Bottom 0.152: BLOW_T_ATT_P.1 13.26,35.05 13.26,35.97 14.78,37.49 14.78,49.38 19.66,54.25 19.66,60.05 R78.2
N$52  (via drill 0.3)
  Top 0.152: v26.36,68.05 32.61,74.3 R63.2
  Bottom 0.152: v26.36,68.05 26.36,52.12 24.69,50.44 24.69,24.69 26.14,23.24 26.14,22.4 STRK_T_P.1
N$53
  Top 0.152: BLOW_T_P.1 13.26,37.64 13.26,38.18 18.52,43.43 18.52,73.15 19.66,74.3 R62.2
N$55
  Bottom 0.152: R77.2 6.78,45.8 6.78,42.98 12.04,37.72 12.04,23.55 13.18,22.4 FLOW_ATT_P.1
N$57
  Bottom 0.152: R81.2 58.67,60.05 58.67,49.99 62.48,46.18 62.48,35.97 64.77,33.68 65.84,33.68 66.45,33.07 66.45,29.41 65.68,28.65 64.77,28.65 64.08,27.96 64.08,20.95 65.23,19.81 DAMP_ATT_P.1
N$58
  Top 0.152: SPCE_ATT_P.1 78.26,24.92 78.26,25.76 82.14,29.64 82.14,44.12 83.44,45.41 83.44,58.9 84.58,60.05 R85.2
N$59
  Top 0.152: LED1.A 46.86,95.25 46.86,82.22 38.94,74.3 38.94,57.45 27.36,45.87 27.36,36.2 26.21,35.05 LED_1.1
N$60
  Top 0.152: LED2.A 46.86,81 46.86,65.53 39.24,57.91 39.24,57.3 27.66,45.72 27.66,33.98 26.21,32.54 LED2_.1
N$62
  Top 0.152: R26.2 71.63,45.8 71.63,39.47 78.18,32.92 78.18,32.54 BRIG_P.1
N$63
  Bottom 0.152: FINE_P.1 65.23,14.78 65.23,15.62 61.87,18.97 61.87,40.84 57.45,45.26 57.45,74.91 61.72,79.17 63.78,79.17 65.3,80.7 65.3,82.3 71.55,88.54 R8.2
N$65
  Top 0.152: GEOM_ATT_P.1 26.21,27.43 26.21,28.35 29.95,32.08 29.95,43.89 31.47,45.41 31.47,46.33 32.16,47.02 44.5,47.02 45.64,45.87 R82.2
N$67
  Top 0.152: R7.2 58.67,88.54 58.67,78.49 64.92,72.24 64.92,41.45 63.09,39.62 63.09,27.05 65.23,24.92 CRSE_P.1
N$68
  Bottom 0.152: FM_P.1 78.18,29.95 78.18,29.11 77.04,27.96 77.04,26.9 77.72,26.21 78.72,26.21 80.16,27.66 80.16,40.08 80.31,40.23 81.69,40.23 81.92,40.46 81.92,44.35 80.92,45.34 80.92,50.6 85.8,55.47 85.8,87.4 84.66,88.54 R9.2
N$69
  Bottom 0.152: STRK_P.1 26.14,24.92 26.14,25.76 24.99,26.9 24.99,46.63 30.18,51.82 30.18,58.45 28.96,59.66 28.96,64.85 31.47,67.36 31.47,87.4 32.61,88.54 R6.2
N$70
  Top 0.152: R24.2 58.67,45.8 58.67,39.47 62.79,35.36 62.79,23.09 64.08,21.79 64.08,18.44 65.23,17.3 GEOM_P.1
N$71
  Top 0.152: MALT_P.1 26.21,17.3 26.21,18.14 30.25,22.17 30.25,43.43 32.61,45.8 R23.2
N$72
  Top 0.152: FLOW_P.1 13.26,32.54 13.26,33.38 19.66,39.78 19.66,45.8 R25.2
N$73
  Top 0.152: R4.2 6.78,88.54 6.78,78.49 13.03,72.24 13.03,42.75 9.37,39.09 9.37,35.74 12.04,33.07 12.04,31.17 13.18,30.02 BOW_P.1
N$74
  Bottom 0.152: R3.2 45.64,25.3 44.81,25.3 40.46,29.64 30.63,29.64 27.36,32.92 27.36,36.42 26.21,37.57 CONT_P.1
N$75
  Top 0.152: R5.2 19.74,88.54 19.74,76.05 21.03,74.75 21.03,33.68 24.69,30.02 24.69,16.23 26.14,14.78 BLOW_P.1
N$76
  Top 0.152: R83.2 71.63,60.05 71.63,47.47 72.92,46.18 72.92,40.31 78.18,35.05 POSI_ATT_P.1
N$77
  Top 0.152: BRIG_ATT_P.1 78.26,22.4 78.26,23.24 82.45,27.43 82.45,43.66 84.58,45.8 R84.2
N$78
  Bottom 0.152: SPCE_P.1 78.26,27.43 78.26,28.27 79.7,29.72 79.7,43.89 78.33,45.26 78.33,68.05 84.58,74.3 R66.2
N$83
  Top 0.152: OUT_R_J.1 83.13,2.21 84.58,2.21 J8.IN
N$85
  Top 0.152: OUT_L_J.1 71.63,3.05 71.63,2.21 J7.IN
N$90
  Bottom 0.152: BOW_T_J.1 12.04,18.44 12.04,21.49 6.78,26.75 6.78,27.66 J9.IN
N$91
  Top 0.152: FLOW_J.1 13.26,14.78 19.58,14.78 19.66,14.86 J10.IN
N$92
  Top 0.152: BLOW_T_J.1 13.26,19.81 13.26,20.73 19.66,27.13 19.66,27.66 J11.IN
N$128
  Top 0.152: SW_LED.1 66.75,28.5 66.75,11.96 65.76,10.97 58.29,10.97 57.91,11.35 45.72,11.35 SW1.L1
SW_GATE
  Top 0.152: SW1.P2 43.2,6.48 48.08,6.48 SW1.P5
  Bottom 0.152: GATE_SW.1 65.3,27.43 65.3,26.59 66.45,25.45 66.45,9.14 65.61,8.31 64.62,8.31 60.88,4.57 49.99,4.57 48.16,6.4 SW1.P5
VCC  (via drill 0.3)
  Top 0.305: v79.93,44.81 75.13,44.81 v73.76,43.43 | v10.21,38.41 10.21,39.17 13.18,42.14 v15.62,42.14 | v29.95,61.87 v25.53,57.45 | v59.51,41.53 v63.63,41.53
  Bottom 0.305: 67.74,39.7 66.67,38.63 66.67,36.42 65.3,35.05 JACK_L.1 | 67.74,39.7 68.05,40.01 68.12,40.01 68.81,40.69 R10.2 68.96,40.77 71.63,43.43 v73.76,43.43 | v79.93,44.81 80.92,43.81 80.92,41.22 R13.2 | v10.21,38.41 7.92,40.69 2.82,40.69 R1.2 | R11.2 15.85,40.92 15.62,41.15 v15.62,42.14 15.7,42.22 15.7,47.62 v25.53,57.45 | 47.93,47.24 48.77,47.24 54.56,41.45 | 47.93,47.24 42.6,47.24 36.12,40.77 30.02,40.77 R2.2 | 54.56,41.45 54.56,40.92 R12.2 | v29.95,61.87 48.39,61.87 49.61,60.66 49.61,55.02 47.93,53.34 47.93,47.24 | 67.74,39.7 65.91,41.53 v63.63,41.53 | v59.51,41.53 54.63,41.53 54.56,41.45

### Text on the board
bPlace: V1.2 | ANTUMBRA | ATOM
tNames: cc-by-sa Olivier Gillet, 2014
